PROGRAM IL
VAR
	RANGE_PG_PS1:RANGEJD;
	RANGE_PG_PS2:RANGEJD;
	RANGE_PG_PS3:RANGEJD;
	RANGE_PG_PS4:RANGEJD;
	RANGE_PG_PS5:RANGEJD;
	RANGE_PG_PS6:RANGEJD;
	RANGE_PG_PS7:RANGEJD;
	RANGE_PG_PS8:RANGEJD;
	RANGE_PG_PS9:RANGEJD;
	
	RANGE_MFC1:RANGEJD;
	RANGE_MFC2:RANGEJD;
	RANGE_MFC3:RANGEJD;
	RANGE_MFC4:RANGEJD;
	RANGE_MFC5:RANGEJD;
	RANGE_MFC6:RANGEJD;
	RANGE_MFC7:RANGEJD;
	RANGE_MFC8:RANGEJD;
	RANGE_MFC9:RANGEJD;
	
	RANGE_CHAMBER_HEATER1:RANGEJD;
	RANGE_CHAMBER_HEATER2:RANGEJD;
	RANGE_CHAMBER_HEATER3:RANGEJD;
	
	RANGE_LID_HEATER:RANGEJD;
	
	RANGE_STAGE_EDGE_HEATER:RANGEJD;
	RANGE_STAGE_CENTER_HEATER:RANGEJD;
	
	//INTERLOCK	
	TON_PrepareTransfer:TON;	
	TON_TransferWafer:TON;	
	TON_OpenGasValve:TON;	
	TON_CloseGasValve:TON;	
	TON_OpenCloseSlitValve:TON;
	
	ALWAYS_TRUE:BOOL:=TRUE;
	VALVE_ITL_BYPASS : ARRAY[1..50] OF BOOL;
	
END_VAR
VAR // added by the converter: edge detectors and wires of the graphical bodies
    _w1, _w2, _w3, _w4, _w5, _w6 : BOOL;
END_VAR

VALVE();
Temp();
SYS();
SPLC();
ACT_HEATER();
ACT_MFC();
ACT_PG_PS();

//TMP Pressure OUT OF RANGE
	IF GV.PMConfig.TurboN2Pressure	<=	GV.TurboN2PurgePressure
		THEN
		PM.INFO.Alarm.TurboN2PurgePressureOutOfRange:=TRUE;
		ELSE
		PM.INFO.Alarm.TurboN2PurgePressureOutOfRange:=FALSE;	
	END_IF
	
//PrepareTransfer TIMEOUT
	TON_PrepareTransfer(IN:= GV_IL.STATUS_PrepareTransfer, PT:=INT_TO_TIME(GV.PMConfig.PrepareTransferTimeout)*1000 , Q=> , ET=> );	
	IF TON_PrepareTransfer.Q
		THEN
		PM.INFO.Alarm.PrepareTransferTimerout:=TRUE;
		ELSE
		PM.INFO.Alarm.PrepareTransferTimerout:=FALSE;
	END_IF
	
//TransferWafer TIMEOUT
	TON_TransferWafer(IN:=GV_IL.STATUS_TransferWafer , PT:= INT_TO_TIME(GV.PMConfig.TransferWaferTimeout)*1000, Q=> , ET=> );
	IF TON_TransferWafer.Q
		THEN
		PM.INFO.Alarm.TransferWaferTimeout:=TRUE;
		ELSE
		PM.INFO.Alarm.TransferWaferTimeout:=FALSE;	
	END_IF
	
//OpenGasValve TIMEOUT
	TON_OpenGasValve(IN:=GV_IL.STATUS_OpenGasValve , PT:= INT_TO_TIME(GV.PMConfig.OpenGasValveTimeout)*1000, Q=> , ET=> );
	IF TON_OpenGasValve.Q
		THEN
		PM.INFO.Alarm.OpenGasValveTimeout:=TRUE;
		ELSE 
		PM.INFO.Alarm.OpenGasValveTimeout:=FALSE;
	END_IF
	
//CloseGasValve TIMEOUT
	TON_CloseGasValve(IN:=GV_IL.STATUS_CloseGasValve , PT:= INT_TO_TIME(GV.PMConfig.CloseGasValveTimeout)*1000, Q=> , ET=> );
	IF TON_CloseGasValve.Q
		THEN
		PM.INFO.Alarm.CloseGasValveTimeout:=TRUE;
		ELSE
		PM.INFO.Alarm.CloseGasValveTimeout:=FALSE;
	END_IF
	
//OpenCloseSlitValve TIMEOUT
	TON_OpenCloseSlitValve(IN:=GV_IL.STATUS_OpenCloseSlitValve , PT:= INT_TO_TIME(GV.PMConfig.OpenCloseSlitValveTimeout)*1000, Q=> , ET=> );
	IF TON_OpenCloseSlitValve.Q
		THEN
		PM.INFO.Alarm.OpenCloseSlitValveTimeout:=TRUE;
		ELSE
		PM.INFO.Alarm.OpenCloseSlitValveTimeout:=FALSE;	
	END_IF
	
	
//PRESSURE ALARM
	//PM.INFO.Alarm.PRESSURE:=
	
//ALARM OR WARNING OCCUR
	GV.ALARM_OCC:=
				 	//PM.INFO.Alarm.PRESSURE
				   PM.INFO.Alarm.MFC1	
				OR PM.INFO.Alarm.MFC2	
				OR PM.INFO.Alarm.MFC3
				OR PM.INFO.Alarm.MFC5	
				OR PM.INFO.Alarm.MFC6
				OR PM.INFO.Alarm.MFC7	
				OR PM.INFO.Alarm.WALL_TEMP	
				OR PM.INFO.Alarm.LID_TEMP	
				OR PM.INFO.Alarm.STAGE_EDGE_TEMP	
				OR PM.INFO.Alarm.STAGE_CENTER_TEMP
				OR PM.INFO.Alarm.Gas1FlowPressureOutOfRange
				OR PM.INFO.Alarm.Gas2FlowPressureOutOfRange
				OR PM.INFO.Alarm.Gas3FlowPressureOutOfRange
				//OR PM.INFO.Alarm.Gas4FlowPressureOutOfRange
				OR PM.INFO.Alarm.Gas5FlowPressureOutOfRange
				OR PM.INFO.Alarm.Gas6FlowPressureOutOfRange
				//OR PM.INFO.Alarm.TurboN2PurgePressureOutOfRange
				//OR PM.INFO.Alarm.PrepareTransferTimerout
				//OR PM.INFO.Alarm.TransferWaferTimeout
				//OR PM.INFO.Alarm.OpenGasValveTimeout
				//OR PM.INFO.Alarm.CloseGasValveTimeout
				//OR PM.INFO.Alarm.OpenCloseSlitValveTimeout
				//OR PM.INFO.Alarm.ATMCheckTimeout
				//OR PM.INFO.Alarm.DRY_PUMP
				//OR PM.INFO.Alarm.PENDULUM_VALVE
				//OR PM.INFO.Alarm.TURBO_PUMP
				OR PM.INFO.Alarm.CHILLER1
				OR PM.INFO.Alarm.CHILLER2
				OR PM.INFO.Alarm.TOLERANCE_PRESSURE				
				OR PM.INFO.Alarm.TOLERANCE_MFC1
				OR PM.INFO.Alarm.TOLERANCE_MFC2
				OR PM.INFO.Alarm.TOLERANCE_MFC3
				OR PM.INFO.Alarm.TOLERANCE_MFC5
				OR PM.INFO.Alarm.TOLERANCE_MFC6
				OR PM.INFO.Alarm.TOLERANCE_MFC7
				OR PM.INFO.Alarm.TOLERANCE_WALL_TEMP
				OR PM.INFO.Alarm.TOLERANCE_LID_TEMP
				OR PM.INFO.Alarm.TOLERANCE_STAGE_EDGE_TEMP
				OR PM.INFO.Alarm.TOLERANCE_STAGE_CENTER_TEMP
				;

	GV.WARNING_OCC:=
					//PM.INFO.Warning.PRESSURE					
					PM.INFO.Warning.MFC1
				OR PM.INFO.Warning.MFC2
				OR PM.INFO.Warning.MFC3
				OR PM.INFO.Warning.MFC5
				OR PM.INFO.Warning.MFC6
				OR PM.INFO.Warning.MFC7
				OR PM.INFO.Warning.WALL_TEMP
				OR PM.INFO.Warning.LID_TEMP
				OR PM.INFO.Warning.STAGE_EDGE_TEMP
				OR PM.INFO.Warning.STAGE_CENTER_TEMP
				OR PM.INFO.Warning.Gas1FlowPressureOutOfRange
				OR PM.INFO.Warning.Gas2FlowPressureOutOfRange
				OR PM.INFO.Warning.Gas3FlowPressureOutOfRange
				//OR PM.INFO.Warning.Gas4FlowPressureOutOfRange
				OR PM.INFO.Warning.Gas5FlowPressureOutOfRange
				OR PM.INFO.Warning.Gas6FlowPressureOutOfRange
				//OR PM.INFO.Warning.OpenCloseSlitValveTimeout
				OR PM.INFO.Warning.CHILLER1
				OR PM.INFO.Warning.CHILLER2
				OR PM.INFO.Warning.TOLERANCE_PRESSURE
				OR PM.INFO.Warning.TOLERANCE_MFC1
				OR PM.INFO.Warning.TOLERANCE_MFC2
				OR PM.INFO.Warning.TOLERANCE_MFC3
				OR PM.INFO.Warning.TOLERANCE_MFC5
				OR PM.INFO.Warning.TOLERANCE_MFC6
				OR PM.INFO.Warning.TOLERANCE_MFC7
				OR PM.INFO.Warning.TOLERANCE_WALL_TEMP
				OR PM.INFO.Warning.TOLERANCE_LID_TEMP
				OR PM.INFO.Warning.TOLERANCE_STAGE_EDGE_TEMP
				OR PM.INFO.Warning.TOLERANCE_STAGE_CENTER_TEMP
				;

ACTION ACT_HEATER:
//CHAMBER HEATER
	RANGE_CHAMBER_HEATER1(
	ENABLE:= GV.ChamberHeater.HeaterTolerance_Enable,
	SV:= REAL_TO_LREAL(GV.AO.Chamber_Temp1_SV),
	PV:= REAL_TO_LREAL( GV.AI.Chamber_Temp1), 
	RANGE_ALARM_H:= ANY_TO_REAL(GV.ChamberHeater.HeaterAlarmRange.SV), 
	RANGE_ALARM_L:= ANY_TO_LREAL(GV.ChamberHeater.HeaterAlarmRange.SV), 
	RANGE_WARNING_H:= ANY_TO_LREAL(GV.ChamberHeater.HeaterWarningRange.SV), 
	RANGE_WARNING_L:= ANY_TO_LREAL(GV.ChamberHeater.HeaterWarningRange.SV), 
	TIME_ALARM:= ANY_TO_LREAL(GV.ChamberHeater.HeaterAlarmTime.SV), 
	TIME_WARNING:= ANY_TO_LREAL(GV.ChamberHeater.HeaterWarningTime.SV), 
	ALARM=> , 
	WARNING=> );
	
	RANGE_CHAMBER_HEATER2(
	ENABLE:= GV.ChamberHeater.HeaterTolerance_Enable,
	SV:= REAL_TO_LREAL(GV.AO.Chamber_Temp2_SV),
	PV:= REAL_TO_LREAL( GV.AI.Chamber_Temp2), 
	RANGE_ALARM_H:= ANY_TO_LREAL(GV.ChamberHeater.HeaterAlarmRange.SV), 
	RANGE_ALARM_L:= ANY_TO_LREAL(GV.ChamberHeater.HeaterAlarmRange.SV), 
	RANGE_WARNING_H:= ANY_TO_LREAL(GV.ChamberHeater.HeaterWarningRange.SV), 
	RANGE_WARNING_L:= ANY_TO_LREAL(GV.ChamberHeater.HeaterWarningRange.SV), 
	TIME_ALARM:= ANY_TO_LREAL(GV.ChamberHeater.HeaterAlarmTime.SV), 
	TIME_WARNING:= ANY_TO_LREAL(GV.ChamberHeater.HeaterWarningTime.SV), 
	ALARM=> , 
	WARNING=> );
	
	RANGE_CHAMBER_HEATER3(
	ENABLE:= GV.ChamberHeater.HeaterTolerance_Enable,
	SV:= REAL_TO_LREAL(GV.AO.Chamber_Temp3_SV),
	PV:= REAL_TO_LREAL( GV.AI.Chamber_Temp3), 
	RANGE_ALARM_H:= ANY_TO_LREAL(GV.ChamberHeater.HeaterAlarmRange.SV), 
	RANGE_ALARM_L:= ANY_TO_LREAL(GV.ChamberHeater.HeaterAlarmRange.SV), 
	RANGE_WARNING_H:= ANY_TO_LREAL(GV.ChamberHeater.HeaterWarningRange.SV), 
	RANGE_WARNING_L:= ANY_TO_LREAL(GV.ChamberHeater.HeaterWarningRange.SV), 
	TIME_ALARM:= ANY_TO_LREAL(GV.ChamberHeater.HeaterAlarmTime.SV), 
	TIME_WARNING:= ANY_TO_LREAL(GV.ChamberHeater.HeaterWarningTime.SV), 
	ALARM=> , 
	WARNING=> );
	
	PM.INFO.Alarm.WALL_TEMP:=	RANGE_CHAMBER_HEATER1.ALARM 
							OR  RANGE_CHAMBER_HEATER2.ALARM 
							OR  RANGE_CHAMBER_HEATER3.ALARM
								;
	PM.INFO.Warning.WALL_TEMP:=	RANGE_CHAMBER_HEATER1.WARNING 
							OR  RANGE_CHAMBER_HEATER2.WARNING 
							OR  RANGE_CHAMBER_HEATER3.WARNING
								;
//LID HEATER
	RANGE_LID_HEATER(
	ENABLE:= GV.LidHeater.HeaterTolerance_Enable,
	SV:= REAL_TO_LREAL(GV.AO.LID_Temp_SV),
	PV:= REAL_TO_LREAL( GV.AI.Lid_Temp), 
	RANGE_ALARM_H:= ANY_TO_LREAL(GV.LidHeater.HeaterAlarmRange.SV), 
	RANGE_ALARM_L:= ANY_TO_LREAL(GV.LidHeater.HeaterAlarmRange.SV), 
	RANGE_WARNING_H:= ANY_TO_LREAL(GV.LidHeater.HeaterWarningRange.SV), 
	RANGE_WARNING_L:= ANY_TO_LREAL(GV.LidHeater.HeaterWarningRange.SV), 
	TIME_ALARM:= ANY_TO_LREAL(GV.LidHeater.HeaterAlarmTime.SV), 
	TIME_WARNING:= ANY_TO_LREAL(GV.LidHeater.HeaterWarningTime.SV), 
	ALARM=> , 
	WARNING=> );
	
	PM.INFO.Alarm.LID_TEMP	:=	RANGE_LID_HEATER.ALARM ;
	PM.INFO.Warning.LID_TEMP:=	RANGE_LID_HEATER.WARNING;
	
//STAGE HEATER
	RANGE_STAGE_CENTER_HEATER(
	ENABLE:= GV.Chiller.EnableAlarmTolerance,
	SV:= REAL_TO_LREAL(GV.AO.Chiller_Temp1_SV),
	PV:= REAL_TO_LREAL( GV.AI.CHILLER1_TEMP_PV), 
	RANGE_ALARM_H:= ANY_TO_LREAL(GV.Chiller.ToleranceAlarmRange.SV), 
	RANGE_ALARM_L:= ANY_TO_LREAL(GV.Chiller.ToleranceAlarmRange.SV), 
	RANGE_WARNING_H:= ANY_TO_LREAL(GV.Chiller.ToleranceAlarmRange.SV), 
	RANGE_WARNING_L:= ANY_TO_LREAL(GV.Chiller.ToleranceAlarmRange.SV), 
	TIME_ALARM:= ANY_TO_LREAL(GV.Chiller.ToleranceAlarmTime.SV), 
	TIME_WARNING:= ANY_TO_LREAL(GV.Chiller.ToleranceAlarmTime.SV), 
	ALARM=> , 
	WARNING=> );
	
	PM.INFO.Alarm.STAGE_CENTER_TEMP:=RANGE_STAGE_CENTER_HEATER.ALARM;
	PM.INFO.Warning.STAGE_CENTER_TEMP:=RANGE_STAGE_CENTER_HEATER.WARNING;
	PM.INFO.Alarm.CHILLER1:= ECC.	CHILLER1_PV.Module2_Word[5].1;
	PM.INFO.Warning.CHILLER1:= ECC.	CHILLER1_PV.Module2_Word[5].2;
	
	RANGE_STAGE_EDGE_HEATER(
	ENABLE:= GV.Chiller.EnableAlarmTolerance,
	SV:= REAL_TO_LREAL(GV.AO.Chiller_Temp2_SV),
	PV:= REAL_TO_LREAL( GV.AI.CHILLER2_TEMP_PV), 
	RANGE_ALARM_H:= ANY_TO_LREAL(GV.Chiller.ToleranceAlarmRange.SV), 
	RANGE_ALARM_L:= ANY_TO_LREAL(GV.Chiller.ToleranceAlarmRange.SV), 
	RANGE_WARNING_H:= ANY_TO_LREAL(GV.Chiller.ToleranceAlarmRange.SV), 
	RANGE_WARNING_L:= ANY_TO_LREAL(GV.Chiller.ToleranceAlarmRange.SV), 
	TIME_ALARM:= ANY_TO_LREAL(GV.Chiller.ToleranceAlarmTime.SV), 
	TIME_WARNING:= ANY_TO_LREAL(GV.Chiller.ToleranceAlarmTime.SV), 
	ALARM=> , 
	WARNING=> );
	
	PM.INFO.Alarm.STAGE_EDGE_TEMP:=RANGE_STAGE_EDGE_HEATER.ALARM;
	PM.INFO.Warning.STAGE_EDGE_TEMP:=RANGE_STAGE_EDGE_HEATER.WARNING;
	PM.INFO.Alarm.CHILLER2:= ECC.	CHILLER2_PV.Module2_Word[5].1;
	PM.INFO.Warning.CHILLER2:= ECC.	CHILLER2_PV.Module2_Word[5].2;
END_ACTION

ACTION ACT_MFC:
RANGE_MFC1(
	ENABLE:= GV.Mfcgas1.EnableAlarm AND GV.Mfcgas1.Enable,
	SV:= REAL_TO_LREAL(GV.AO.MFC1_Flow_Setpoint),
	PV:= REAL_TO_LREAL( GV.AI.MFC1_Flow), 
	RANGE_ALARM_H:= GV.Mfcgas1.AlarmRange.SV, 
	RANGE_ALARM_L:= GV.Mfcgas1.AlarmRange.SV, 
	RANGE_WARNING_H:= GV.Mfcgas1.WarningRange.SV, 
	RANGE_WARNING_L:= GV.Mfcgas1.WarningRange.SV, 
	TIME_ALARM:= GV.Mfcgas1.AlarmTime.SV, 
	TIME_WARNING:= GV.Mfcgas1.WarningTime.SV, 
	ALARM=> , 
	WARNING=> );
	
	RANGE_MFC2(
	ENABLE:= GV.Mfcgas2.EnableAlarm AND GV.Mfcgas2.Enable, 
	SV:= REAL_TO_LREAL(GV.AO.MFC2_Flow_Setpoint),
	PV:= REAL_TO_LREAL( GV.AI.MFC2_Flow), 
	RANGE_ALARM_H:= GV.Mfcgas2.AlarmRange.SV, 
	RANGE_ALARM_L:= GV.Mfcgas2.AlarmRange.SV, 
	RANGE_WARNING_H:= GV.Mfcgas2.WarningRange.SV, 
	RANGE_WARNING_L:= GV.Mfcgas2.WarningRange.SV, 
	TIME_ALARM:= GV.Mfcgas2.AlarmTime.SV, 
	TIME_WARNING:= GV.Mfcgas2.WarningTime.SV, 
	ALARM=> , 
	WARNING=> );

	RANGE_MFC3(	
	ENABLE:= GV.Mfcgas3.EnableAlarm AND GV.Mfcgas3.Enable, 
	SV:= REAL_TO_LREAL(GV.AO.MFC3_Flow_Setpoint),
	PV:= REAL_TO_LREAL( GV.AI.MFC3_Flow), 
	RANGE_ALARM_H:= GV.Mfcgas3.AlarmRange.SV, 
	RANGE_ALARM_L:= GV.Mfcgas3.AlarmRange.SV, 
	RANGE_WARNING_H:= GV.Mfcgas3.WarningRange.SV, 
	RANGE_WARNING_L:= GV.Mfcgas3.WarningRange.SV, 
	TIME_ALARM:= GV.Mfcgas3.AlarmTime.SV, 
	TIME_WARNING:= GV.Mfcgas3.WarningTime.SV,  
	ALARM=> , 
	WARNING=> );
(*
	RANGE_MFC4(	
	ENABLE:= GV.Mfcgas4.EnableAlarm AND GV.Mfcgas4.Enable, 
	SV:= REAL_TO_LREAL(GV.AO.MFC4_Flow_Setpoint),
	PV:= REAL_TO_LREAL( GV.AI.MFC4_Flow), 
	RANGE_ALARM_H:= GV.Mfcgas4.AlarmRange.SV, 
	RANGE_ALARM_L:= GV.Mfcgas4.AlarmRange.SV, 
	RANGE_WARNING_H:= GV.Mfcgas4.WarningRange.SV, 
	RANGE_WARNING_L:= GV.Mfcgas4.WarningRange.SV, 
	TIME_ALARM:= GV.Mfcgas4.AlarmTime.SV, 
	TIME_WARNING:= GV.Mfcgas4.WarningTime.SV, 
	ALARM=> , 
	WARNING=> );
*)	
	RANGE_MFC5(	
	ENABLE:= GV.Mfcgas5.EnableAlarm AND GV.Mfcgas5.Enable, 
	SV:= REAL_TO_LREAL(GV.AO.MFC5_Flow_Setpoint),
	PV:= REAL_TO_LREAL( GV.AI.MFC5_Flow), 
	RANGE_ALARM_H:= GV.Mfcgas5.AlarmRange.SV, 
	RANGE_ALARM_L:= GV.Mfcgas5.AlarmRange.SV, 
	RANGE_WARNING_H:= GV.Mfcgas5.WarningRange.SV, 
	RANGE_WARNING_L:= GV.Mfcgas5.WarningRange.SV, 
	TIME_ALARM:= GV.Mfcgas5.AlarmTime.SV, 
	TIME_WARNING:= GV.Mfcgas5.WarningTime.SV, 
	ALARM=> , 
	WARNING=> );

	RANGE_MFC6(	
	ENABLE:= GV.Mfcgas6.EnableAlarm AND GV.Mfcgas6.Enable, 
	SV:= REAL_TO_LREAL(GV.AO.MFC6_Flow_Setpoint),
	PV:= REAL_TO_LREAL( GV.AI.MFC6_Flow), 
	RANGE_ALARM_H:= GV.Mfcgas6.AlarmRange.SV, 
	RANGE_ALARM_L:= GV.Mfcgas6.AlarmRange.SV, 
	RANGE_WARNING_H:= GV.Mfcgas6.WarningRange.SV, 
	RANGE_WARNING_L:= GV.Mfcgas6.WarningRange.SV, 
	TIME_ALARM:= GV.Mfcgas6.AlarmTime.SV, 
	TIME_WARNING:= GV.Mfcgas6.WarningTime.SV,  
	ALARM=> , 
	WARNING=> );

	RANGE_MFC7(	
	ENABLE:= GV.Mfcgas7.EnableAlarm AND GV.Mfcgas7.Enable, 
	SV:= REAL_TO_LREAL(GV.AO.MFC7_Flow_Setpoint),
	PV:= REAL_TO_LREAL( GV.AI.MFC7_Flow), 
	RANGE_ALARM_H:= GV.Mfcgas7.AlarmRange.SV, 
	RANGE_ALARM_L:= GV.Mfcgas7.AlarmRange.SV, 
	RANGE_WARNING_H:= GV.Mfcgas7.WarningRange.SV, 
	RANGE_WARNING_L:= GV.Mfcgas7.WarningRange.SV, 
	TIME_ALARM:= GV.Mfcgas7.AlarmTime.SV, 
	TIME_WARNING:= GV.Mfcgas7.WarningTime.SV, 
	ALARM=> , 
	WARNING=> );
(*
	RANGE_MFC8(	
	ENABLE:= GV.Mfcgas8.EnableAlarm AND GV.Mfcgas8.Enable, 
	PV:= REAL_TO_LREAL( GV.AI.MFC8_Flow), 
	RANGE_ALARM_H:= GV.Mfcgas8.AlarmRange.MaxSV, 
	RANGE_ALARM_L:= 0, 
	RANGE_WARNING_H:= GV.Mfcgas8.WarningRange.MaxSV, 
	RANGE_WARNING_L:= 0, 
	TIME_ALARM:= GV.Mfcgas8.AlarmTime.SV, 
	TIME_WARNING:= GV.Mfcgas8.WarningTime.SV, 
	ALARM=> , 
	WARNING=> );

	RANGE_MFC9(	
	ENABLE:= GV.Mfcgas9.EnableAlarm AND GV.Mfcgas9.Enable, 
	PV:= REAL_TO_LREAL( GV.AI.MFC9_Flow), 
	RANGE_ALARM_H:= GV.Mfcgas9.AlarmRange.MaxSV, 
	RANGE_ALARM_L:= 0, 
	RANGE_WARNING_H:= GV.Mfcgas9.WarningRange.MaxSV, 
	RANGE_WARNING_L:= 0, 
	TIME_ALARM:= GV.Mfcgas9.AlarmTime.SV, 
	TIME_WARNING:= GV.Mfcgas9.WarningTime.SV, 
	ALARM=> , 
	WARNING=> );
*)	
	
	PM.Info.Alarm.MFC1:=  RANGE_MFC1.ALARM;
	PM.INFO.Alarm.MFC2:=  RANGE_MFC2.ALARM;
	PM.INFO.Alarm.MFC3:=  RANGE_MFC3.ALARM;
//	PM.INFO.Alarm.MFC4:=  RANGE_MFC4.ALARM;
	PM.INFO.Alarm.MFC5:=  RANGE_MFC5.ALARM;
	PM.INFO.Alarm.MFC6:=  RANGE_MFC6.ALARM;
	PM.INFO.Alarm.MFC7:=  RANGE_MFC7.ALARM;
//	PM.INFO.Alarm.MFC8:=  RANGE_MFC8.ALARM;
//	PM.INFO.Alarm.MFC9:=  RANGE_MFC9.ALARM;
	
	PM.INFO.warning.MFC1:=  RANGE_MFC1.warning;
	PM.INFO.warning.MFC2:=  RANGE_MFC2.warning;
	PM.INFO.warning.MFC3:=  RANGE_MFC3.warning;
//	PM.INFO.warning.MFC4:=  RANGE_MFC4.warning;
	PM.INFO.warning.MFC5:=  RANGE_MFC5.warning;
	PM.INFO.warning.MFC6:=  RANGE_MFC6.warning;
	PM.INFO.warning.MFC7:=  RANGE_MFC7.warning;
//	PM.INFO.warning.MFC8:=  RANGE_MFC8.warning;
//	PM.INFO.warning.MFC9:=  RANGE_MFC9.warning;
END_ACTION

ACTION ACT_PG_PS:
RANGE_PG_PS1(
	ENABLE:=TRUE,
	SV:= 270,
	PV:= GV.AI.PG_PS1_VALUE, 
	RANGE_ALARM_H:= GV.PMConfig.GasFlowPressureAlarmRange, 
	RANGE_ALARM_L:= GV.PMConfig.GasFlowPressureAlarmRange, 
	RANGE_WARNING_H:= GV.PMConfig.GasFlowPressureWarningRange, 
	RANGE_WARNING_L:= GV.PMConfig.GasFlowPressureWarningRange, 
	TIME_ALARM:= GV.PMConfig.GasFlowPressureAlarmTime, 
	TIME_WARNING:= GV.PMConfig.GasFlowPressureWarningTime, 
	ALARM=> , 
	WARNING=> );
	
	RANGE_PG_PS2(
	ENABLE:=TRUE,
	SV:= 270 ,
	PV:= GV.AI.PG_PS2_VALUE, 
	RANGE_ALARM_H:= GV.PMConfig.GasFlowPressureAlarmRange, 
	RANGE_ALARM_L:= GV.PMConfig.GasFlowPressureAlarmRange, 
	RANGE_WARNING_H:= GV.PMConfig.GasFlowPressureWarningRange, 
	RANGE_WARNING_L:= GV.PMConfig.GasFlowPressureWarningRange, 
	TIME_ALARM:= GV.PMConfig.GasFlowPressureAlarmTime, 
	TIME_WARNING:= GV.PMConfig.GasFlowPressureWarningTime, 
	ALARM=> , 
	WARNING=> );
	
	RANGE_PG_PS3(
	ENABLE:=TRUE,
	SV:= 270 ,
	PV:= GV.AI.PG_PS3_VALUE, 
	RANGE_ALARM_H:= GV.PMConfig.GasFlowPressureAlarmRange, 
	RANGE_ALARM_L:= GV.PMConfig.GasFlowPressureAlarmRange, 
	RANGE_WARNING_H:= GV.PMConfig.GasFlowPressureWarningRange, 
	RANGE_WARNING_L:= GV.PMConfig.GasFlowPressureWarningRange, 
	TIME_ALARM:= GV.PMConfig.GasFlowPressureAlarmTime, 
	TIME_WARNING:= GV.PMConfig.GasFlowPressureWarningTime, 
	ALARM=> , 
	WARNING=> );
	
	RANGE_PG_PS4(
	ENABLE:=TRUE,
	SV:=25,
	PV:= GV.AI.PG_PS4_VALUE, 
	RANGE_ALARM_H:= GV.PMConfig.GasFlowPressureAlarmRange, 
	RANGE_ALARM_L:= GV.PMConfig.GasFlowPressureAlarmRange, 
	RANGE_WARNING_H:= GV.PMConfig.GasFlowPressureWarningRange, 
	RANGE_WARNING_L:= GV.PMConfig.GasFlowPressureWarningRange, 
	TIME_ALARM:= GV.PMConfig.GasFlowPressureAlarmTime, 
	TIME_WARNING:= GV.PMConfig.GasFlowPressureWarningTime, 
	ALARM=> , 
	WARNING=> );
	
	RANGE_PG_PS5(
	ENABLE:=TRUE,
	SV:= 270,
	PV:= GV.AI.PG_PS5_VALUE, 
	RANGE_ALARM_H:= GV.PMConfig.GasFlowPressureAlarmRange, 
	RANGE_ALARM_L:= GV.PMConfig.GasFlowPressureAlarmRange, 
	RANGE_WARNING_H:= GV.PMConfig.GasFlowPressureWarningRange, 
	RANGE_WARNING_L:= GV.PMConfig.GasFlowPressureWarningRange, 
	TIME_ALARM:= GV.PMConfig.GasFlowPressureAlarmTime, 
	TIME_WARNING:= GV.PMConfig.GasFlowPressureWarningTime, 
	ALARM=> , 
	WARNING=> );
	
	RANGE_PG_PS6(
	ENABLE:=TRUE,
	SV:=270,
	PV:= GV.AI.PG_PS6_VALUE, 
	RANGE_ALARM_H:= GV.PMConfig.GasFlowPressureAlarmRange, 
	RANGE_ALARM_L:= GV.PMConfig.GasFlowPressureAlarmRange, 
	RANGE_WARNING_H:= GV.PMConfig.GasFlowPressureWarningRange, 
	RANGE_WARNING_L:= GV.PMConfig.GasFlowPressureWarningRange, 
	TIME_ALARM:= GV.PMConfig.GasFlowPressureAlarmTime, 
	TIME_WARNING:= GV.PMConfig.GasFlowPressureWarningTime, 
	ALARM=> , 
	WARNING=> );
(*	
	RANGE_PG_PS7(
	ENABLE:=TRUE,
	PV:= GV.AI.PG_PS7_VALUE, 
	RANGE_ALARM_H:= GV.PMConfig.GasFlowPressureAlarmRange, 
	RANGE_ALARM_L:= GV.PMConfig.GasFlowPressureAlarmRange, 
	RANGE_WARNING_H:= GV.PMConfig.GasFlowPressureWarningRange, 
	RANGE_WARNING_L:= GV.PMConfig.GasFlowPressureWarningRange, 
	TIME_ALARM:= GV.PMConfig.GasFlowPressureAlarmTime, 
	TIME_WARNING:= GV.PMConfig.GasFlowPressureWarningTime, 
	ALARM=> , 
	WARNING=> );
	
	RANGE_PG_PS8(
	ENABLE:=TRUE,
	PV:= GV.AI.PG_PS8_VALUE, 
	RANGE_ALARM_H:= GV.PMConfig.GasFlowPressureAlarmRange, 
	RANGE_ALARM_L:= GV.PMConfig.GasFlowPressureAlarmRange, 
	RANGE_WARNING_H:= GV.PMConfig.GasFlowPressureWarningRange, 
	RANGE_WARNING_L:= GV.PMConfig.GasFlowPressureWarningRange, 
	TIME_ALARM:= GV.PMConfig.GasFlowPressureAlarmTime, 
	TIME_WARNING:= GV.PMConfig.GasFlowPressureWarningTime, 
	ALARM=> , 
	WARNING=> );
	
	RANGE_PG_PS9(
	ENABLE:=TRUE,
	PV:= GV.AI.PG_PS9_VALUE, 
	RANGE_ALARM_H:= GV.PMConfig.GasFlowPressureAlarmRange, 
	RANGE_ALARM_L:= GV.PMConfig.GasFlowPressureAlarmRange, 
	RANGE_WARNING_H:= GV.PMConfig.GasFlowPressureWarningRange, 
	RANGE_WARNING_L:= GV.PMConfig.GasFlowPressureWarningRange, 
	TIME_ALARM:= GV.PMConfig.GasFlowPressureAlarmTime, 
	TIME_WARNING:= GV.PMConfig.GasFlowPressureWarningTime, 
	ALARM=> , 
	WARNING=> );
*)	
	PM.INFO.Alarm.Gas1FlowPressureOutOfRange:=  RANGE_PG_PS1.ALARM;
	PM.INFO.Alarm.Gas2FlowPressureOutOfRange:=  RANGE_PG_PS2.ALARM;
	PM.INFO.Alarm.Gas3FlowPressureOutOfRange:=  RANGE_PG_PS3.ALARM;	
	PM.INFO.Alarm.Gas4FlowPressureOutOfRange:=  RANGE_PG_PS4.ALARM;
	PM.INFO.Alarm.Gas5FlowPressureOutOfRange:=  RANGE_PG_PS5.ALARM;
	PM.INFO.Alarm.Gas6FlowPressureOutOfRange:=  RANGE_PG_PS6.ALARM;
	//PM.INFO.Alarm.Gas7FlowPressureOutOfRange:=  RANGE_PG_PS7.ALARM;
	//PM.INFO.Alarm.Gas8FlowPressureOutOfRange:=  RANGE_PG_PS8.ALARM;
	//PM.INFO.Alarm.Gas9FlowPressureOutOfRange:=  RANGE_PG_PS9.ALARM;

	PM.INFO.warning.Gas1FlowPressureOutOfRange:=  RANGE_PG_PS1.warning;
	PM.INFO.warning.Gas2FlowPressureOutOfRange:=  RANGE_PG_PS2.warning;
	PM.INFO.warning.Gas3FlowPressureOutOfRange:=  RANGE_PG_PS3.warning;
	PM.INFO.warning.Gas4FlowPressureOutOfRange:=  RANGE_PG_PS4.warning;
	PM.INFO.warning.Gas5FlowPressureOutOfRange:=  RANGE_PG_PS5.warning;
	PM.INFO.warning.Gas6FlowPressureOutOfRange:=  RANGE_PG_PS6.warning;
	//PM.INFO.warning.Gas7FlowPressureOutOfRange:=  RANGE_PG_PS7.warning;
	//PM.INFO.warning.Gas8FlowPressureOutOfRange:=  RANGE_PG_PS8.warning;
	//PM.INFO.warning.Gas9FlowPressureOutOfRange:=  RANGE_PG_PS9.warning;
END_ACTION

ACTION SPLC:
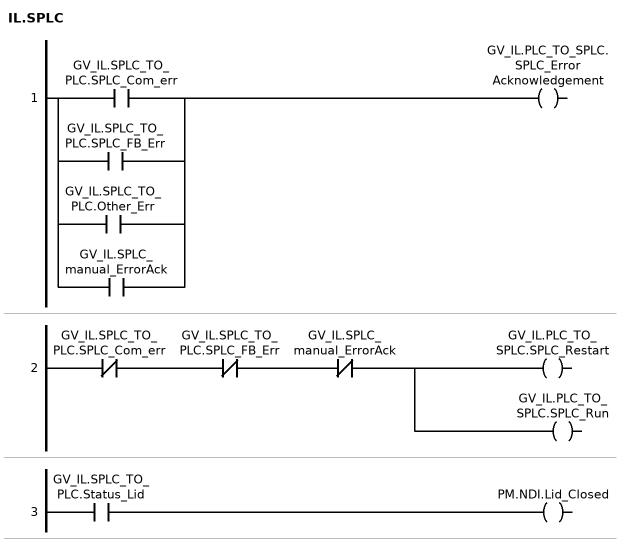
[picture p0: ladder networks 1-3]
// NETWORK 1
GV_IL.PLC_TO_SPLC.SPLC_ErrorAcknowledgement := GV_IL.SPLC_TO_PLC.SPLC_Com_err OR GV_IL.SPLC_TO_PLC.SPLC_FB_Err OR GV_IL.SPLC_TO_PLC.Other_Err OR GV_IL.SPLC_manual_ErrorAck;

// NETWORK 2
_w1 := NOT GV_IL.SPLC_TO_PLC.SPLC_Com_err AND NOT GV_IL.SPLC_TO_PLC.SPLC_FB_Err AND NOT GV_IL.SPLC_manual_ErrorAck;
GV_IL.PLC_TO_SPLC.SPLC_Restart := _w1;
GV_IL.PLC_TO_SPLC.SPLC_Run := _w1;

// NETWORK 3
PM.NDI.Lid_Closed := GV_IL.SPLC_TO_PLC.Status_Lid;
END_ACTION

ACTION SYS:
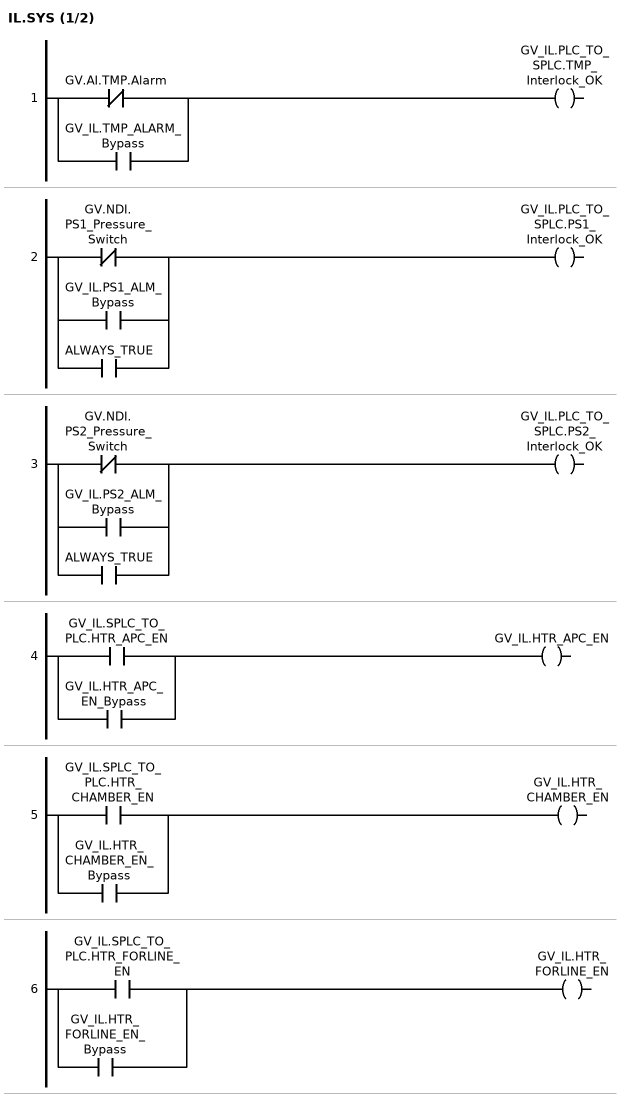
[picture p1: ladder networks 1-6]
// NETWORK 1
GV_IL.PLC_TO_SPLC.TMP_Interlock_OK := NOT GV.AI.TMP.Alarm OR GV_IL.TMP_ALARM_Bypass;

// NETWORK 2
GV_IL.PLC_TO_SPLC.PS1_Interlock_OK := NOT (GV.NDI.	PS1_Pressure_Switch) OR GV_IL.PS1_ALM_Bypass OR ALWAYS_TRUE;

// NETWORK 3
GV_IL.PLC_TO_SPLC.PS2_Interlock_OK := NOT (GV.NDI.	PS2_Pressure_Switch) OR GV_IL.PS2_ALM_Bypass OR ALWAYS_TRUE;

// NETWORK 4
GV_IL.HTR_APC_EN := GV_IL.SPLC_TO_PLC.HTR_APC_EN OR GV_IL.HTR_APC_EN_Bypass;

// NETWORK 5
GV_IL.HTR_CHAMBER_EN := GV_IL.SPLC_TO_PLC.HTR_CHAMBER_EN OR GV_IL.HTR_CHAMBER_EN_Bypass;

// NETWORK 6
GV_IL.HTR_FORLINE_EN := GV_IL.SPLC_TO_PLC.HTR_FORLINE_EN OR GV_IL.HTR_FORLINE_EN_Bypass;

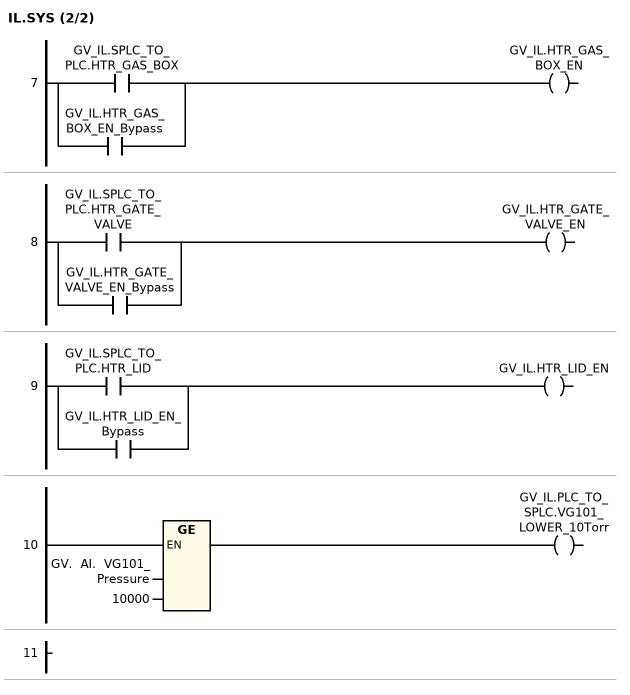
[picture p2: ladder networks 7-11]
// NETWORK 7
GV_IL.HTR_GAS_BOX_EN := GV_IL.SPLC_TO_PLC.HTR_GAS_BOX OR GV_IL.HTR_GAS_BOX_EN_Bypass;

// NETWORK 8
GV_IL.HTR_GATE_VALVE_EN := GV_IL.SPLC_TO_PLC.HTR_GATE_VALVE OR GV_IL.HTR_GATE_VALVE_EN_Bypass;

// NETWORK 9
GV_IL.HTR_LID_EN := GV_IL.SPLC_TO_PLC.HTR_LID OR GV_IL.HTR_LID_EN_Bypass;

// NETWORK 10
GV_IL.PLC_TO_SPLC.VG101_LOWER_10Torr := (GV.	AI.	VG101_Pressure) >= 10000;

// NETWORK 11
END_ACTION

ACTION Temp:
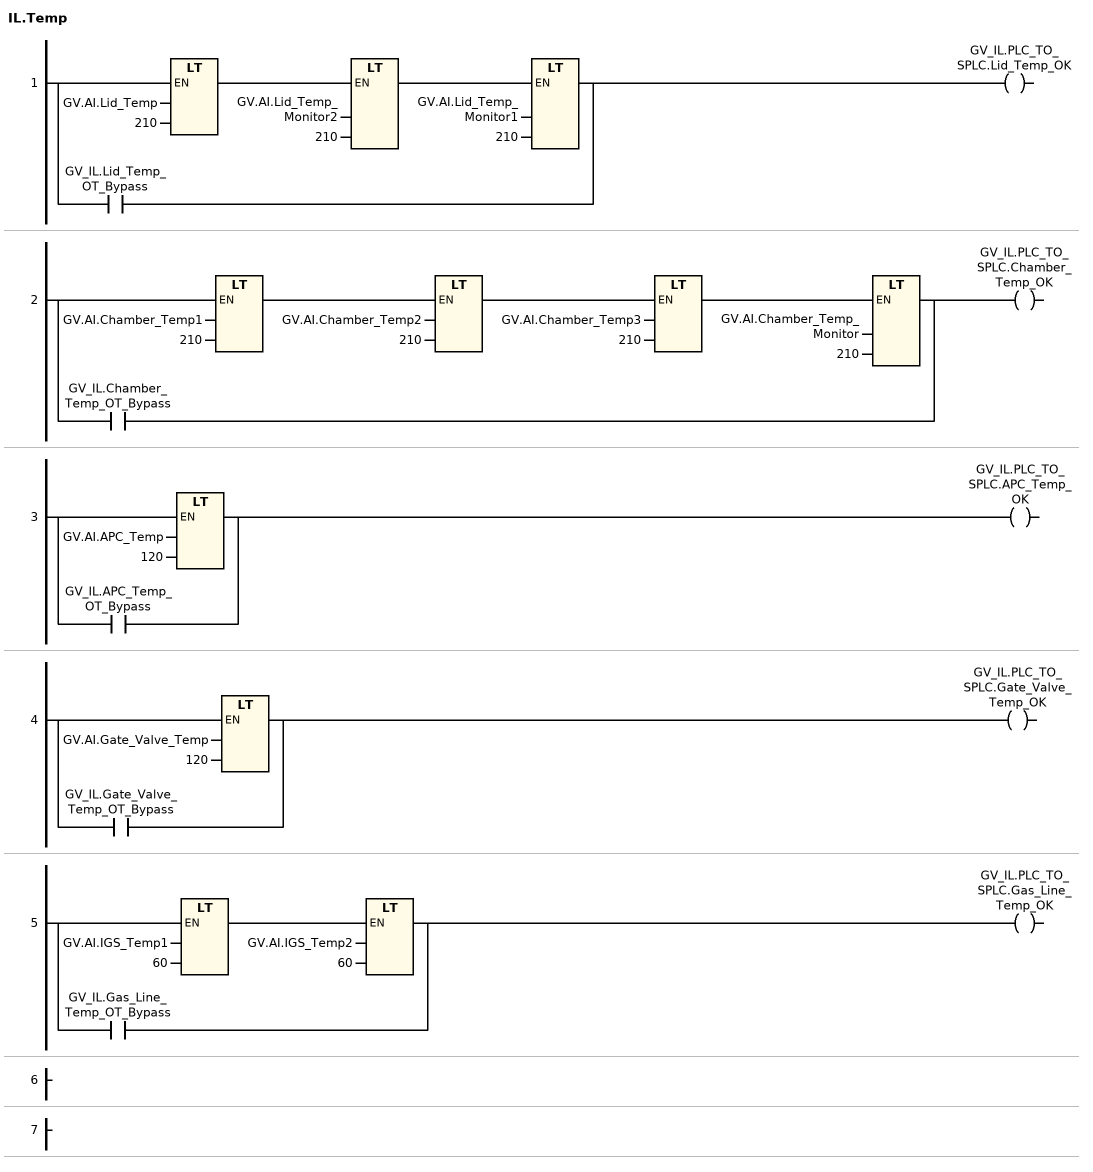
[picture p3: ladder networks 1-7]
// NETWORK 1
_w2 := GV_IL.Lid_Temp_OT_Bypass;
IF NOT _w2 THEN
    _w2 := GV.AI.Lid_Temp < 210 AND GV.AI.Lid_Temp_Monitor2 < 210 AND GV.AI.Lid_Temp_Monitor1 < 210;
END_IF
GV_IL.PLC_TO_SPLC.Lid_Temp_OK := _w2;

// NETWORK 2
_w3 := GV_IL.Chamber_Temp_OT_Bypass;
IF NOT _w3 THEN
    _w3 := GV.AI.Chamber_Temp1 < 210 AND GV.AI.Chamber_Temp2 < 210 AND GV.AI.Chamber_Temp3 < 210 AND GV.AI.Chamber_Temp_Monitor < 210;
END_IF
GV_IL.PLC_TO_SPLC.Chamber_Temp_OK := _w3;

// NETWORK 3
_w4 := GV_IL.APC_Temp_OT_Bypass;
IF NOT _w4 THEN
    _w4 := GV.AI.APC_Temp < 120;
END_IF
GV_IL.PLC_TO_SPLC.APC_Temp_OK := _w4;

// NETWORK 4
_w5 := GV_IL.Gate_Valve_Temp_OT_Bypass;
IF NOT _w5 THEN
    _w5 := GV.AI.Gate_Valve_Temp < 120;
END_IF
GV_IL.PLC_TO_SPLC.Gate_Valve_Temp_OK := _w5;

// NETWORK 5
_w6 := GV_IL.Gas_Line_Temp_OT_Bypass;
IF NOT _w6 THEN
    _w6 := GV.AI.IGS_Temp1 < 60 AND GV.AI.IGS_Temp2 < 60;
END_IF
GV_IL.PLC_TO_SPLC.Gas_Line_Temp_OK := _w6;

// NETWORK 6

// NETWORK 7
END_ACTION

ACTION TM:
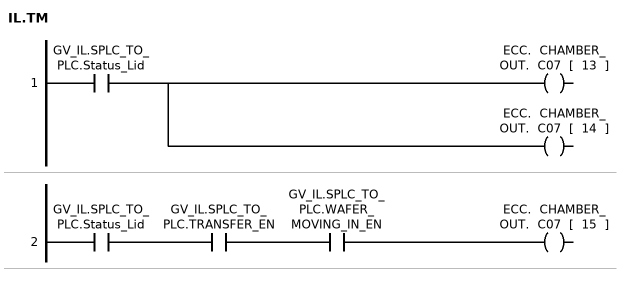
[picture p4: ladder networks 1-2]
// NETWORK 1
ECC.	CHAMBER_OUT.	C07	[	13	] := GV_IL.SPLC_TO_PLC.Status_Lid;
ECC.	CHAMBER_OUT.	C07	[	14	] := GV_IL.SPLC_TO_PLC.Status_Lid;

// NETWORK 2
ECC.	CHAMBER_OUT.	C07	[	15	] := GV_IL.SPLC_TO_PLC.Status_Lid AND GV_IL.SPLC_TO_PLC.TRANSFER_EN AND GV_IL.SPLC_TO_PLC.WAFER_MOVING_IN_EN;
END_ACTION

ACTION VALVE:
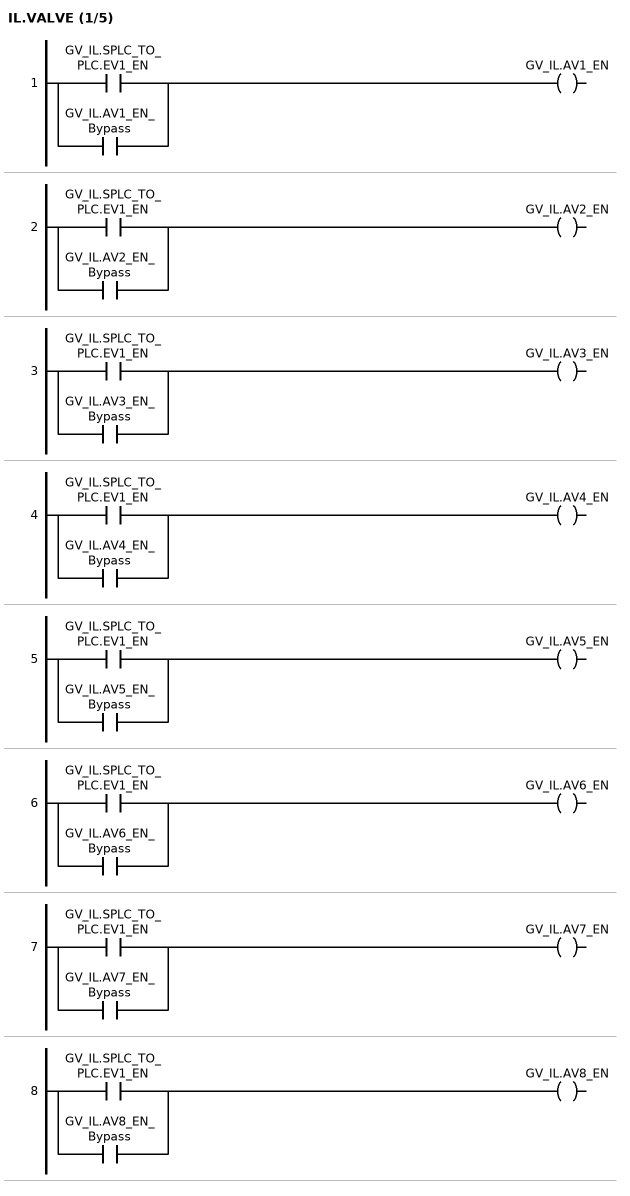
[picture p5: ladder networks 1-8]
// NETWORK 1
GV_IL.AV1_EN := GV_IL.SPLC_TO_PLC.EV1_EN OR GV_IL.AV1_EN_Bypass;

// NETWORK 2
GV_IL.AV2_EN := GV_IL.SPLC_TO_PLC.EV1_EN OR GV_IL.AV2_EN_Bypass;

// NETWORK 3
GV_IL.AV3_EN := GV_IL.SPLC_TO_PLC.EV1_EN OR GV_IL.AV3_EN_Bypass;

// NETWORK 4
GV_IL.AV4_EN := GV_IL.SPLC_TO_PLC.EV1_EN OR GV_IL.AV4_EN_Bypass;

// NETWORK 5
GV_IL.AV5_EN := GV_IL.SPLC_TO_PLC.EV1_EN OR GV_IL.AV5_EN_Bypass;

// NETWORK 6
GV_IL.AV6_EN := GV_IL.SPLC_TO_PLC.EV1_EN OR GV_IL.AV6_EN_Bypass;

// NETWORK 7
GV_IL.AV7_EN := GV_IL.SPLC_TO_PLC.EV1_EN OR GV_IL.AV7_EN_Bypass;

// NETWORK 8
GV_IL.AV8_EN := GV_IL.SPLC_TO_PLC.EV1_EN OR GV_IL.AV8_EN_Bypass;

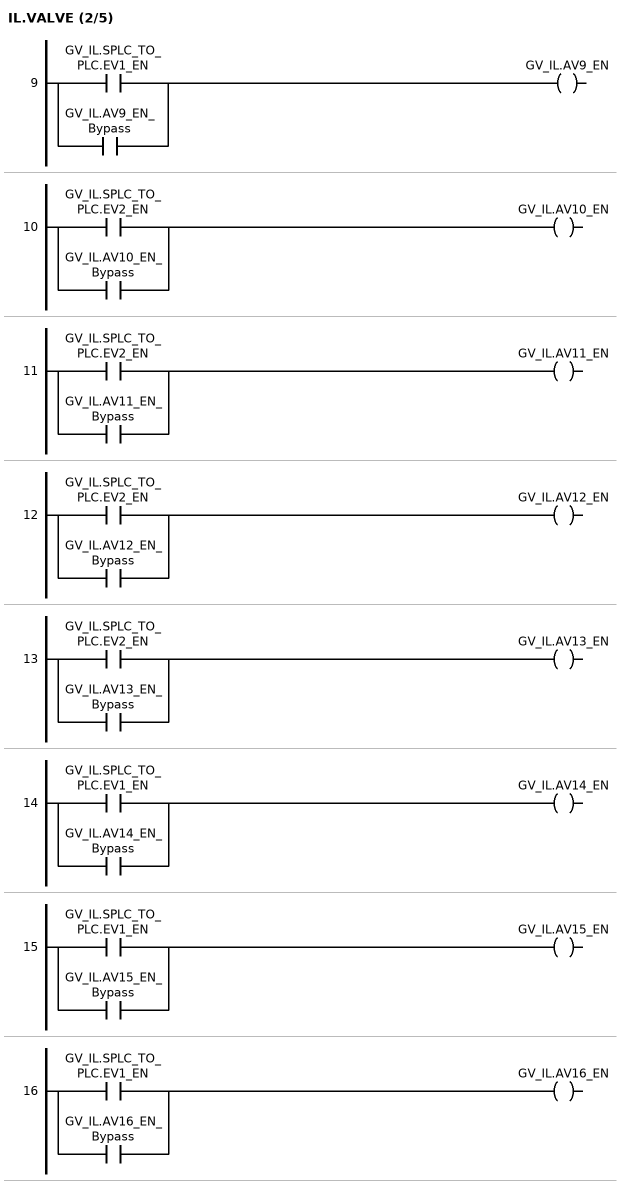
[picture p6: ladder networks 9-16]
// NETWORK 9
GV_IL.AV9_EN := GV_IL.SPLC_TO_PLC.EV1_EN OR GV_IL.AV9_EN_Bypass;

// NETWORK 10
GV_IL.AV10_EN := GV_IL.SPLC_TO_PLC.EV2_EN OR GV_IL.AV10_EN_Bypass;

// NETWORK 11
GV_IL.AV11_EN := GV_IL.SPLC_TO_PLC.EV2_EN OR GV_IL.AV11_EN_Bypass;

// NETWORK 12
GV_IL.AV12_EN := GV_IL.SPLC_TO_PLC.EV2_EN OR GV_IL.AV12_EN_Bypass;

// NETWORK 13
GV_IL.AV13_EN := GV_IL.SPLC_TO_PLC.EV2_EN OR GV_IL.AV13_EN_Bypass;

// NETWORK 14
GV_IL.AV14_EN := GV_IL.SPLC_TO_PLC.EV1_EN OR GV_IL.AV14_EN_Bypass;

// NETWORK 15
GV_IL.AV15_EN := GV_IL.SPLC_TO_PLC.EV1_EN OR GV_IL.AV15_EN_Bypass;

// NETWORK 16
GV_IL.AV16_EN := GV_IL.SPLC_TO_PLC.EV1_EN OR GV_IL.AV16_EN_Bypass;

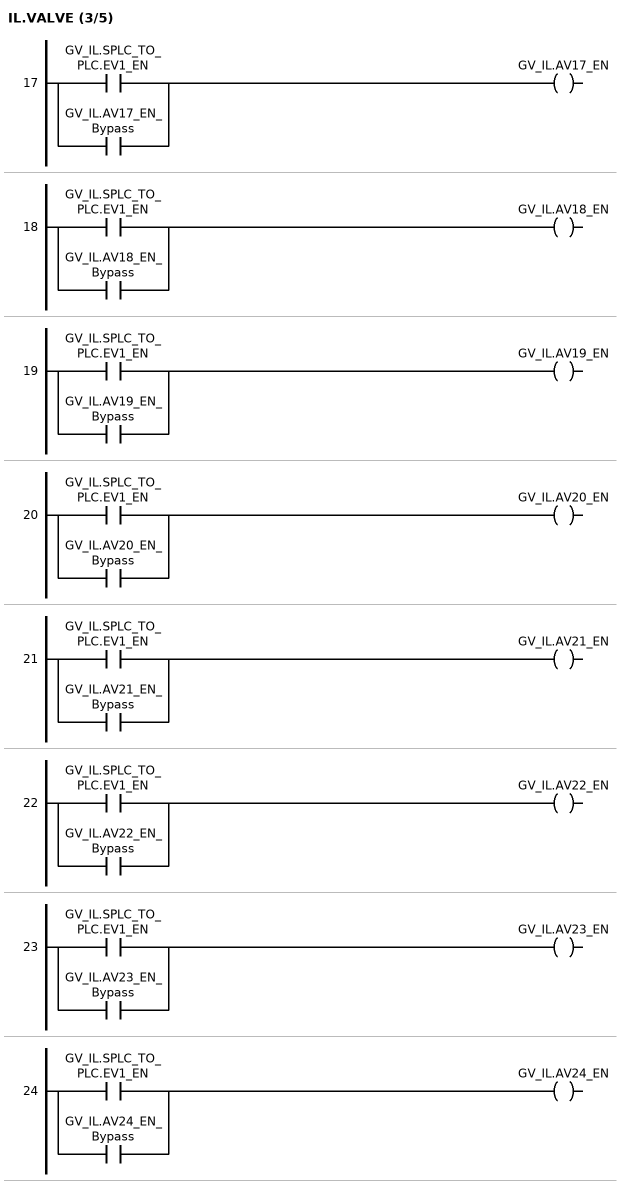
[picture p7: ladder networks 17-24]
// NETWORK 17
GV_IL.AV17_EN := GV_IL.SPLC_TO_PLC.EV1_EN OR GV_IL.AV17_EN_Bypass;

// NETWORK 18
GV_IL.AV18_EN := GV_IL.SPLC_TO_PLC.EV1_EN OR GV_IL.AV18_EN_Bypass;

// NETWORK 19
GV_IL.AV19_EN := GV_IL.SPLC_TO_PLC.EV1_EN OR GV_IL.AV19_EN_Bypass;

// NETWORK 20
GV_IL.AV20_EN := GV_IL.SPLC_TO_PLC.EV1_EN OR GV_IL.AV20_EN_Bypass;

// NETWORK 21
GV_IL.AV21_EN := GV_IL.SPLC_TO_PLC.EV1_EN OR GV_IL.AV21_EN_Bypass;

// NETWORK 22
GV_IL.AV22_EN := GV_IL.SPLC_TO_PLC.EV1_EN OR GV_IL.AV22_EN_Bypass;

// NETWORK 23
GV_IL.AV23_EN := GV_IL.SPLC_TO_PLC.EV1_EN OR GV_IL.AV23_EN_Bypass;

// NETWORK 24
GV_IL.AV24_EN := GV_IL.SPLC_TO_PLC.EV1_EN OR GV_IL.AV24_EN_Bypass;

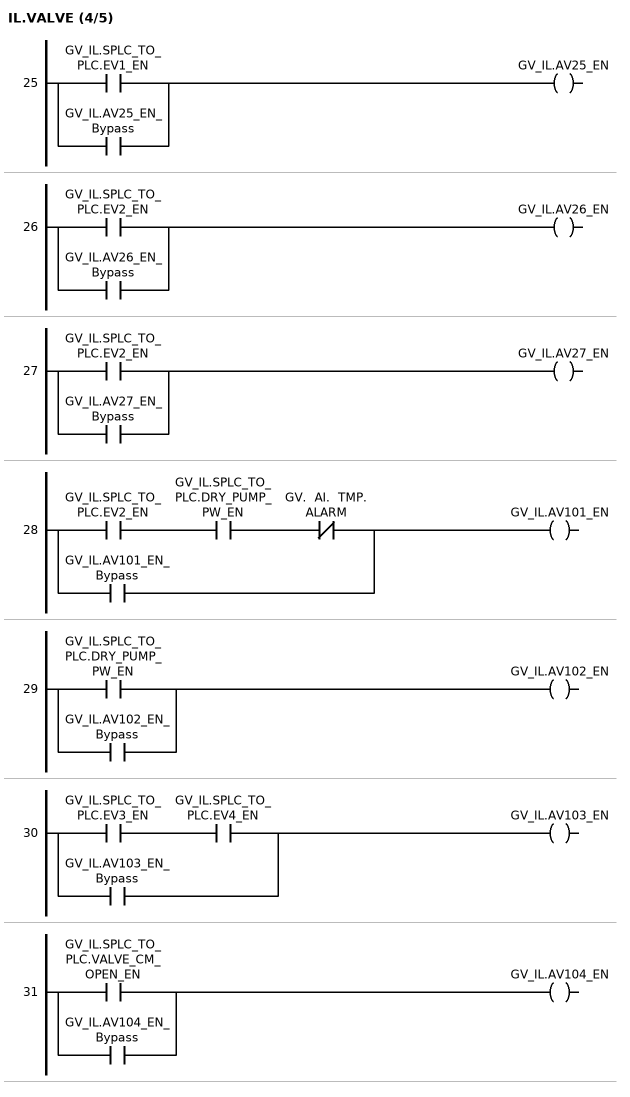
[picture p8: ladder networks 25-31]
// NETWORK 25
GV_IL.AV25_EN := GV_IL.SPLC_TO_PLC.EV1_EN OR GV_IL.AV25_EN_Bypass;

// NETWORK 26
GV_IL.AV26_EN := GV_IL.SPLC_TO_PLC.EV2_EN OR GV_IL.AV26_EN_Bypass;

// NETWORK 27
GV_IL.AV27_EN := GV_IL.SPLC_TO_PLC.EV2_EN OR GV_IL.AV27_EN_Bypass;

// NETWORK 28
GV_IL.AV101_EN := GV_IL.SPLC_TO_PLC.EV2_EN AND GV_IL.SPLC_TO_PLC.DRY_PUMP_PW_EN AND NOT (GV.	AI.	TMP.	ALARM) OR GV_IL.AV101_EN_Bypass;

// NETWORK 29
GV_IL.AV102_EN := GV_IL.SPLC_TO_PLC.DRY_PUMP_PW_EN OR GV_IL.AV102_EN_Bypass;

// NETWORK 30
GV_IL.AV103_EN := GV_IL.SPLC_TO_PLC.EV3_EN AND GV_IL.SPLC_TO_PLC.EV4_EN OR GV_IL.AV103_EN_Bypass;

// NETWORK 31
GV_IL.AV104_EN := GV_IL.SPLC_TO_PLC.VALVE_CM_OPEN_EN OR GV_IL.AV104_EN_Bypass;

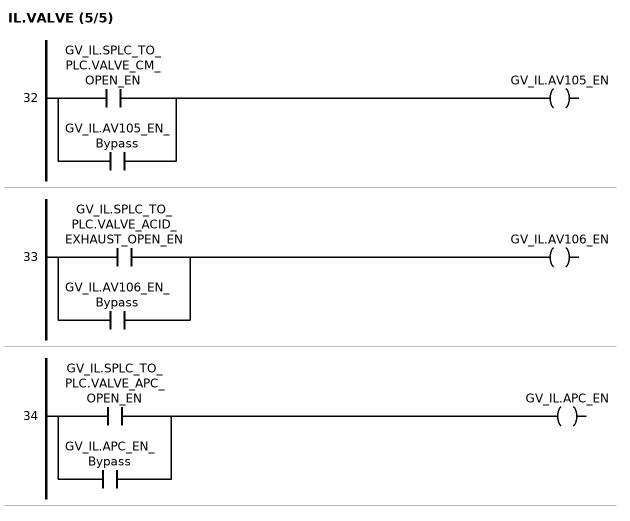
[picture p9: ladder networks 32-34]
// NETWORK 32
GV_IL.AV105_EN := GV_IL.SPLC_TO_PLC.VALVE_CM_OPEN_EN OR GV_IL.AV105_EN_Bypass;

// NETWORK 33
GV_IL.AV106_EN := GV_IL.SPLC_TO_PLC.VALVE_ACID_EXHAUST_OPEN_EN OR GV_IL.AV106_EN_Bypass;

// NETWORK 34
GV_IL.APC_EN := GV_IL.SPLC_TO_PLC.VALVE_APC_OPEN_EN OR GV_IL.APC_EN_Bypass;
END_ACTION

END_PROGRAM
